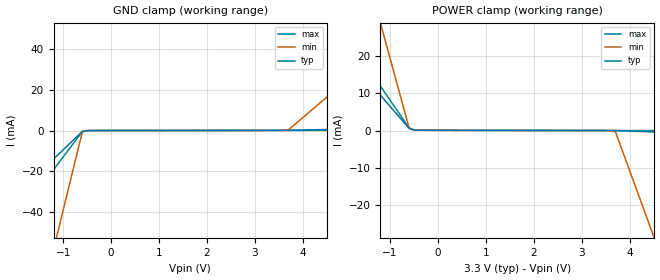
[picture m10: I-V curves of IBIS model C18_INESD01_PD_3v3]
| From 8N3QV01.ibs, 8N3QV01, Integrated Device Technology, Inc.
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[Model] C18_INESD01_PD_3v3
Model_type   Input
Polarity   Non-Inverting
Vinl = 0.8V
Vinh = 2.0V
|   typ   min   max
C_comp   2pF   1.5pF   2.5pF
|   typ   min   max
[Voltage range]   3.3V   3.135V   3.465V
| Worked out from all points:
|   GND clamp passes 1 mA (typ) near -0.62 V on its own axis
|   POWER clamp passes 1 mA (typ) near -0.63 V on its own axis
[GND_clamp]
|Voltage   I (typ)   I (min)   I (max)
-3.3V     -61.32mA   -259.6mA   -84.4mA
-2.9V     -52.31mA   -221.3mA   -71.97mA
-2.8V     -50.05mA   -211.7mA   -68.87mA
-2.3V     -38.78mA   -163.7mA   -53.33mA
-2.2V     -36.52mA   -154.1mA   -50.23mA
-1.2V     -13.98mA   -58.24mA   -19.17mA
-1.1V     -11.73mA   -48.65mA   -16.06mA
-600mV    -453.3uA   -698.6uA   -527.7uA
-400mV    -11.1uA    -13uA      -9.761uA
3.7V      77.31uA    339.6uA    78.55uA
6.2V      1.427mA    50.43mA    134.4uA
6.6V      1.643mA    58.44mA    143.4uA
[Power_clamp]
|Voltage   I (typ)   I (min)   I (max)
-3.3V     40.74mA    127.9mA    51.33mA
-2.5V     28.83mA    90.18mA    36.32mA
-2.4V     27.35mA    85.47mA    34.44mA
-2.1V     22.88mA    71.33mA    28.82mA
-2V       21.4mA     66.62mA    26.94mA
-1.2V     9.494mA    28.91mA    11.94mA
-1.1V     8.006mA    24.2mA     10.06mA
-600mV    567.9uA    633.8uA    683uA
-500mV    131.3uA    131.4uA    134.2uA
3.7V      -11.1uA    -299.6uA   -4.991uA
4.5V      -367.9uA   -28.5mA    -22.78uA
6.6V      -1.304mA   -102.5mA   -69.48uA
